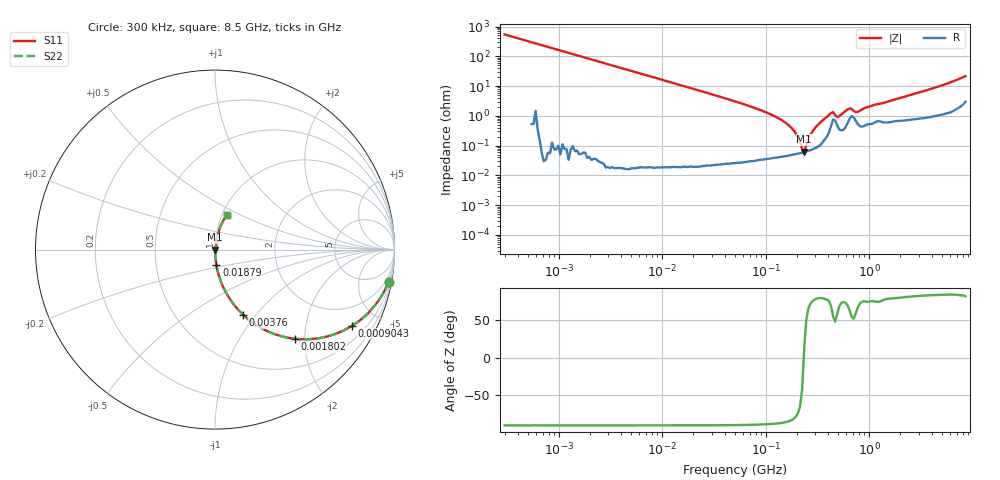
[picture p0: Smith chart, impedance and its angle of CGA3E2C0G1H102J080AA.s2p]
! S-parameter Generated by TDK Corporation
! Copyright(C) 2015 TDK Corporation.
! All Rights Reserved.
! TDK P/N: CGA3E2C0G1H102J080AA (Multilayer Ceramic Chip Capacitors)
! Property: C=1nF
! Size(LxWxT): 1.6x0.8x0.8mm, 0.063x0.031x0.031inches
! Model Type: s2p (Touchstone File Format Version 1.0)
! Frequency: DC=Yes Start=0.3MHz Stop=8500MHz 225points Log-sweep
! Note:
! Model Generated on Jun. 23, 2015
! Hash(MD5):
! Port Assignments:
!  1 ---| |--- 2
! Applicable Conditions:
!  Temperature = 25 degC
!  DC Bias Voltage = 0 V
!  Small Signal Operation
! Terms and conditions regarding TDK Simulation Models
! (1)This simulation model is being provided solely for informational purposes. Please refer to the specifications of the products in terms of detailed characteristics of such products.
! (2)In no event shall TDK Corporation of any of its subsidiaries be liable for any loss or damage arising, directly or indirectly,
!  From any information contained in this simulation model, including, but not limited to loss or damages arising from any inaccuracies, omissions or errors in connection with such information.
! (3)Any and all copyrights on this simulation model are owned by TDK Corporation.
!  Duplication or redistribution of this simulation model without prior written permission from TDK Corporation is prohibited.
! (4)This simulation model is subject to any modification or change without any prior notice.
! (5)Neither TDK Corporation nor any of its subsidiaries shall make any warranty, express or implied,
!  Including but not limited to the correctness, implied warranties of merchantability and fitness for a particular purpose with respect to this simulation models.
! (6)The use of this simulation model shall be deemed to have consented to the terms and conditions hereof.
# MHz S MA R 50
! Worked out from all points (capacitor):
!   224 points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, 300 kHz to 8.5 GHz, reference 50 ohm
!   read as one part in series: C = 984 pF near 314.1 kHz
!   lowest |Z| = 63.4 mohm at 235.6 MHz (marker M1)
!   series resonance near 233.3 MHz, so ESL is about 470 pH
!   S11 on the Smith chart (normalised r, x): 300 kHz: 1, -11; 904.3 kHz: 1.00, -3.59; 1.802 MHz: 1.00, -1.80; 3.76 MHz: 1.00, -0.86; 18.79 MHz: 1.00, -0.17; 8.5 GHz: 1.06, +0.43
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0.3  0.9833 -10.5  0.1821 79.5  0.1821 79.5  0.9833 -10.5
0.9042579  0.8732 -29.1  0.487 60.8  0.487 60.8  0.8732 -29.1
1.72111  0.6855 -46.7  0.7276 43.3  0.7276 43.3  0.6855 -46.7
1.802081  0.6687 -48.0  0.7431 42.0  0.7431 42.0  0.6687 -48.0
3.760292  0.396 -66.6  0.9181 23.3  0.9181 23.3  0.396 -66.6
9.430415  0.1693 -80.2  0.9854 9.7  0.9854 9.7  0.1693 -80.2
18.79372  0.08546 -85.0  0.9961 4.9  0.9961 4.9  0.08546 -85.0
51.67171  0.02985 -87.8  0.9993 1.7  0.9993 1.7  0.02985 -87.8
102.9757  0.01271 -87.7  0.9996 0.7  0.9996 0.7  0.01271 -87.7
155.7485  0.005841 -85.3  0.9995 0.3  0.9995 0.3  0.005841 -85.3
195.9978  0.002532 -78.0  0.9995 0.1  0.9995 0.1  0.002532 -78.0
224.9819  0.0007698 -41.4  0.9994 0.0  0.9994 0.0  0.0007698 -41.4
235.5662  0.000633 12.8  0.9994 -0.0  0.9994 -0.0  0.000633 12.8
258.2521  0.001624 65.5  0.9993 -0.1  0.9993 -0.1  0.001624 65.5
283.1228  0.002987 75.4  0.9993 -0.2  0.9993 -0.2  0.002987 75.4
428.2171  0.01255 68.0  0.9954 -0.7  0.9954 -0.7  0.01255 68.0
448.3627  0.01311 54.3  0.9924 -0.6  0.9924 -0.6  0.01311 54.3
491.5417  0.009031 58.2  0.9953 -0.4  0.9953 -0.4  0.009031 58.2
647.669  0.0175 62.0  0.9919 -0.9  0.9919 -0.9  0.0175 62.0
743.4462  0.01316 59.0  0.9933 -0.7  0.9933 -0.7  0.01316 59.0
1551.304  0.03086 77.0  0.9935 -1.7  0.9935 -1.7  0.03086 77.0
8500  0.2049 70.3  0.9508 -11.7  0.9508 -11.7  0.2049 70.3
